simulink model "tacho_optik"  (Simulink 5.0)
settings: Solver=ode4  StartTime=0.0  StopTime=2  FixedStep=0.0001  RelTol=1e-6

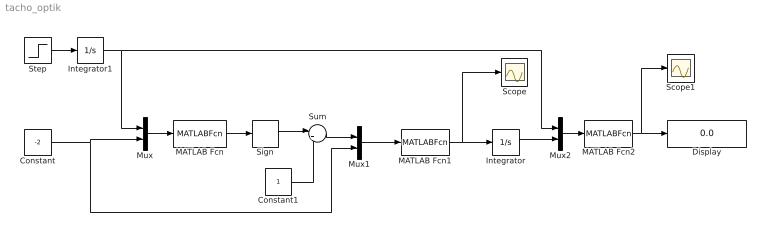
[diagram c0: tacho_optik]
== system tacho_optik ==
  Constant : Constant  Value=-2
  Constant1 : Constant
  Display : Display
  Integrator : Integrator
  Integrator1 : Integrator
  MATLAB Fcn : MATLABFcn  MATLABFcn=optik
  MATLAB Fcn1 : MATLABFcn  MATLABFcn=arah_putaran
  MATLAB Fcn2 : MATLABFcn  MATLABFcn=perata
  Mux : Mux  Inputs=2
  Mux1 : Mux  Inputs=2
  Mux2 : Mux  Inputs=2
  Scope : Scope
  Scope1 : Scope
  Sign : Signum
  Step : Step  Time=0  SampleTime=0
  Sum : Sum  Inputs=|++
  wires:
  Constant/1 -> Mux/2, Mux1/2
  Step/1 -> Integrator1/1
  Integrator1/1 -> Mux/1, Mux2/1
  Mux/1 -> MATLAB Fcn/1
  MATLAB Fcn/1 -> Sign/1
  Sign/1 -> Sum/1
  Constant1/1 -> Sum/2
  MATLAB Fcn1/1 -> Integrator/1, Scope/1
  Sum/1 -> Mux1/1
  Mux1/1 -> MATLAB Fcn1/1
  Integrator/1 -> Mux2/2
  Mux2/1 -> MATLAB Fcn2/1
  MATLAB Fcn2/1 -> Display/1, Scope1/1
